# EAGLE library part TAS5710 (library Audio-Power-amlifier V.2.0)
Texas Instruments, The TAS5710 is a 20-W, efficient, digital audio power amplifier for driving stereo bridge-tied speakers. A 32-bit datapath eliminates the need for pre-scaling before processing and preserves signal integrity without sacrificing dynamic range. A digital audio processor with fully programmable digital filters allows designers to custom tune speakers for optimum sound in small enclosures. A programmable DRC can adjust power levels for a scaleable design while also enabling night-mode listening modes.
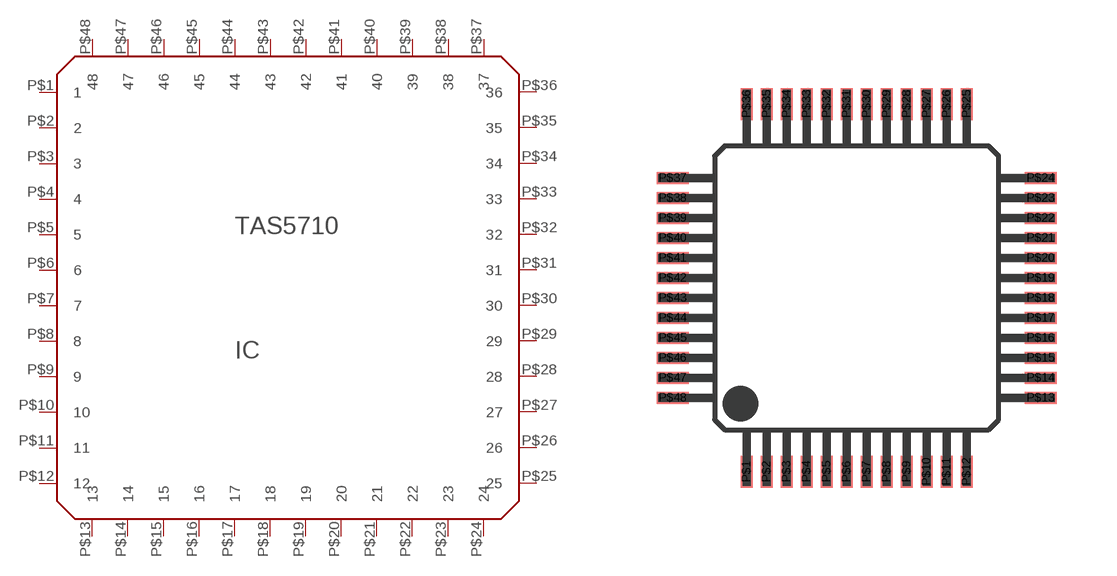
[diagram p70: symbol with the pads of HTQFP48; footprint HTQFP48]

Designator prefix IC

## TAS5710  [HTQFP48]
P$1  1  out
P$2  2  pwr
P$3  3  pwr
P$4  4  out
P$5  5  pwr
P$6  6  pwr
P$7  7  pwr
P$8  8  pwr
P$9  9  pwr
P$10  10
P$11  11
P$12  12
P$13  13  pwr
P$14  14
P$15  15
P$16  16
P$17  17
P$18  18
P$19  19
P$20  20
P$21  21
P$22  22
P$23  23
P$24  24
P$25  25
P$26  26
P$27  27  pwr
P$28  28  pwr
P$29  29  pwr
P$30  30  pwr
P$31  31  pwr
P$32  32  pwr
P$33  33  out
P$34  34  pwr
P$35  35  pwr
P$36  36  out
P$37  37  pwr
P$38  38
P$39  39
P$40  40
P$41  41
P$42  42  pwr
P$43  43  pwr
P$44  44
P$45  45
P$46  46
P$47  47
P$48  48  pwr

## Footprint HTQFP48 (pad centres in mm)
smd 0.3 x 0.8: P$1 -2.75,-4.6; P$2 -2.25,-4.6; P$3 -1.75,-4.6; P$4 -1.25,-4.6; P$5 -0.75,-4.6; P$6 -0.25,-4.6; P$7 0.25,-4.6; P$8 0.75,-4.6; P$9 1.25,-4.6; P$10 1.75,-4.6; P$11 2.25,-4.6; P$12 2.75,-4.6; P$25 2.75,4.6; P$26 2.25,4.6; P$27 1.75,4.6; P$28 1.25,4.6; P$29 0.75,4.6; P$30 0.25,4.6; P$31 -0.25,4.6; P$32 -0.75,4.6; P$33 -1.25,4.6; P$34 -1.75,4.6; P$35 -2.25,4.6; P$36 -2.75,4.6
smd 0.8 x 0.3: P$13 4.6,-2.75; P$14 4.6,-2.25; P$15 4.6,-1.75; P$16 4.6,-1.25; P$17 4.6,-0.75; P$18 4.6,-0.25; P$19 4.6,0.25; P$20 4.6,0.75; P$21 4.6,1.25; P$22 4.6,1.75; P$23 4.6,2.25; P$24 4.6,2.75; P$37 -4.6,2.75; P$38 -4.6,2.25; P$39 -4.6,1.75; P$40 -4.6,1.25; P$41 -4.6,0.75; P$42 -4.6,0.25; P$43 -4.6,-0.25; P$44 -4.6,-0.75; P$45 -4.6,-1.25; P$46 -4.6,-1.75; P$47 -4.6,-2.25; P$48 -4.6,-2.75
